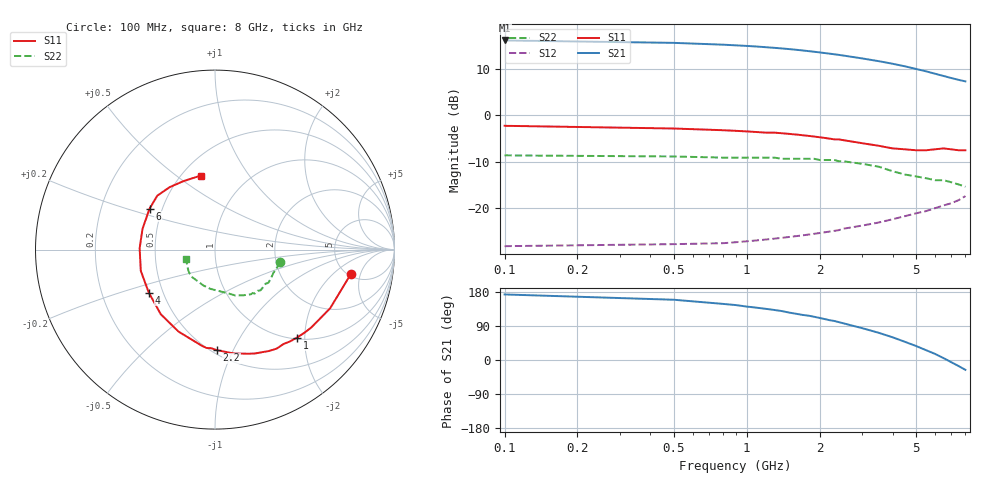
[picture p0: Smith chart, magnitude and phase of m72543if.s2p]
!  MGA-72543 S PARAMETERS
!  Vd=3V  Id=60 mA Vc=0.1V  LAST UPDATED 01-27-99
# ghz s ma r 50
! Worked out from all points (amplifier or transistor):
!   31 points, 100 MHz to 8 GHz, reference 50 ohm
!   highest |S21| = 16.1 dB at 100 MHz (marker M1)
!   |S21| within 3 dB of that: start of sweep to 2.32 GHz
!   unconditionally stable (mu >= 1): start of sweep to end of sweep
!   at 1.1 GHz: K = 1.27, MAG = 17.8 dB, |S12| = -26.9 dB
!   at 2.1 GHz: K = 1.34, MAG = 15.8 dB, |S12| = -25.2 dB
!   at 8 GHz: K = 1.37, MAG = 8.7 dB, |S12| = -17.4 dB
!   lowest NFmin = 1.46 dB at 900 MHz
!   S11 on the Smith chart (normalised r, x): 100 MHz: 5.34, -3.51; 1 GHz: 1.03, -1.83; 2.2 GHz: 0.53, -0.87; 4 GHz: 0.42, -0.25; 6 GHz: 0.43, +0.24; 8 GHz: 0.62, +0.62
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0.1  0.77 -10.0  6.383 173.0  0.039 17.0  0.37 -11.0
0.5  0.72 -27.0  6.013 159.0  0.041 10.0  0.36 -16.0
0.8  0.69 -39.0  5.748 148.0  0.042 13.0  0.35 -22.0
0.9  0.68 -43.0  5.657 145.0  0.043 14.0  0.35 -24.0
1  0.67 -47.0  5.575 141.0  0.044 15.0  0.35 -26.0
1.2  0.65 -54.0  5.4 135.0  0.046 17.0  0.35 -30.0
1.4  0.64 -62.0  5.233 129.0  0.048 18.0  0.34 -34.0
1.6  0.62 -69.0  5.068 122.0  0.05 19.0  0.34 -38.0
1.9  0.59 -79.0  4.824 114.0  0.053 20.0  0.34 -42.0
2.2  0.56 -89.0  4.602 105.0  0.056 20.0  0.33 -46.0
2.3  0.55 -92.0  4.532 103.0  0.057 20.0  0.33 -48.0
2.5  0.54 -98.0  4.395 97.0  0.06 19.0  0.32 -51.0
3  0.5 -114.0  4.089 84.0  0.065 18.0  0.3 -58.0
3.5  0.47 -130.0  3.825 72.0  0.07 17.0  0.28 -66.0
4  0.44 -147.0  3.585 60.0  0.076 15.0  0.25 -75.0
4.5  0.43 -164.0  3.363 48.0  0.082 12.0  0.23 -86.0
5  0.42 179.0  3.153 37.0  0.088 9.0  0.22 -97.0
5.5  0.42 164.0  2.972 26.0  0.093 6.0  0.21 -108.0
6  0.43 148.0  2.796 16.0  0.1 3.0  0.2 -121.0
6.5  0.44 137.0  2.647 5.0  0.107 -1.0  0.2 -132.0
7  0.43 126.0  2.514 -6.0  0.113 -5.0  0.19 -141.0
8  0.42 101.0  2.316 -26.0  0.135 -14.0  0.17 -162.0
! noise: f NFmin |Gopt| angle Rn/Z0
0.8  1.61  0.43  36  0.41
1  1.51  0.46  40  0.39
1.8  1.81  0.35  64  0.33
2  1.85  0.33  71  0.31
2.2  1.86  0.32  77  0.3
2.4  1.89  0.32  84  0.28
3  1.95  0.3  103  0.24
4  2.02  0.29  143  0.16
5  2.13  0.32  -178  0.13
6  2.23  0.38  -138  0.18
